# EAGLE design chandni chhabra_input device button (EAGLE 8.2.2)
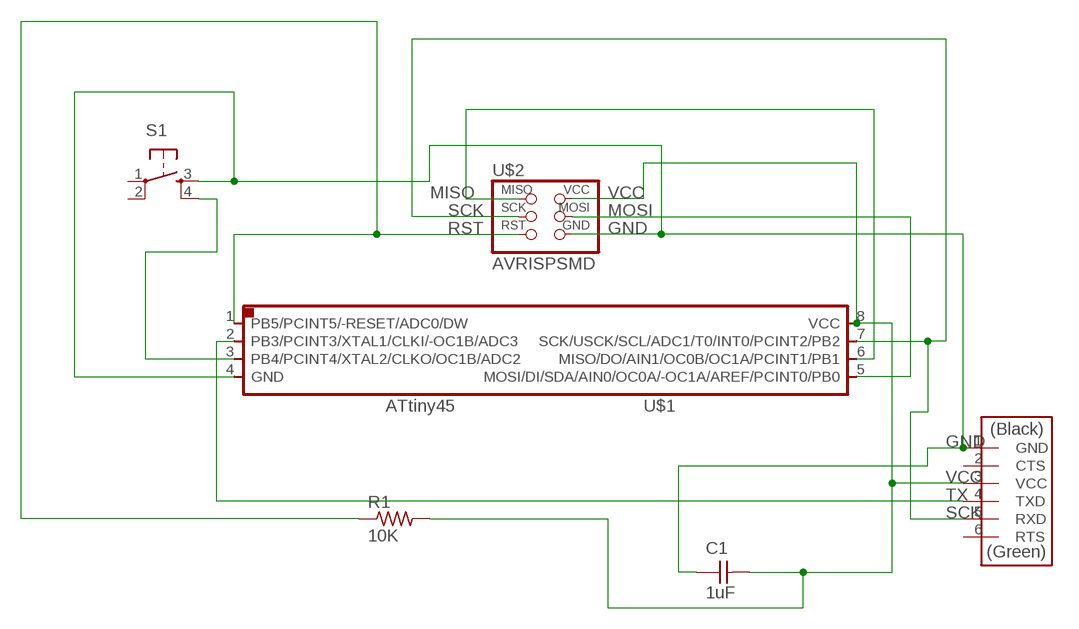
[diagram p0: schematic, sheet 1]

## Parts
C1  1uF  CAP-UNPOLARIZEDFAB  [C1206FAB]
R1  10K  RES-US1206FAB  [R1206FAB]
S1  6MM_SWITCH6MM_SWITCH  [6MM_SWITCH]
U$1  ATTINY45SI  [SOIC8]
U$2  AVRISPSMD  [2X03SMD]
U$3  FTDI-SMD-HEADER  [1X06SMD]

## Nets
GND: C1.1 S1.3(S) U$1.4(GND) U$2.6(GND) U$3.1(GND)
MISO: U$1.6(MISO/DO/AIN1/OC0B/OC1A/PCINT1/PB1) U$2.1(MISO)
MOSI: U$1.5(MOSI/DI/SDA/AIN0/OC0A/-OC1A/AREF/PCINT0/PB0) U$2.4(MOSI)
N$1: S1.4(S1) U$1.3(PB4/PCINT4/XTAL2/CLKO/OC1B/ADC2)
RST: R1.1 U$1.1(PB5/PCINT5/-RESET/ADC0/DW) U$2.5(RST)
SCK: U$1.7(SCK/USCK/SCL/ADC1/T0/INT0/PCINT2/PB2) U$2.3(SCK) U$3.5(RXD)
TX: U$1.2(PB3/PCINT3/XTAL1/CLKI/-OC1B/ADC3) U$3.4(TXD)
VCC: C1.2 R1.2 U$1.8(VCC) U$2.2(VCC) U$3.3(VCC)
Unconnected: S1.1(P) S1.2(P1) U$3.2(CTS) U$3.6(RTS)

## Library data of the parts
C1 = fab:CAP-UNPOLARIZED
R1 = fab:RES-US: Resistor (US Symbol)
S1 = fab:6MM_SWITCH: OMRON SWITCH
U$1 = fab:ATTINY45
U$2 = fab:AVRISP
U$3 = fab:FTDI-SMD-HEADER

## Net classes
0 default: width 0.32 mm, clearance 0.4 mm

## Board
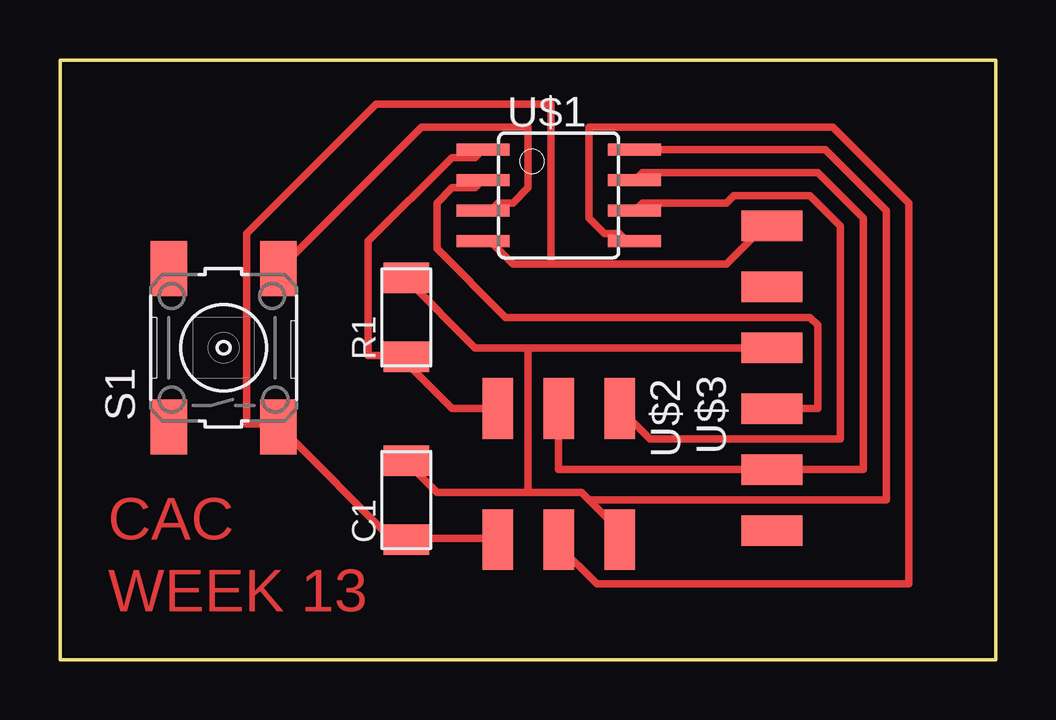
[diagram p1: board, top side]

Size 39 x 25 mm. Coordinates in mm from the lower left corner, seen from the top.
Outline: 39,25 0,25 0,0 39,0 39,25
Copper layers (1*16): Top 0.035mm / dielectric 1.5mm / Bottom 0.035mm
Design rules "fab": minimum track width 0.3mm, minimum drill 32mil, track to track 0.315mm, track to pad 0.315mm, pad to pad 0.315mm, via to via 0.315mm, smd to smd 0.315mm, copper to edge 40mil, drill to drill 16mil, minimum pad ring 10mil, minimum via ring 8mil, stop-mask expansion 4mil, vias tented up to drill 0mil, thermal gap 10mil

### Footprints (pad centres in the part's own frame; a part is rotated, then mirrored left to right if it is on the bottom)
C1206FAB = smd 1.27 x 1.905: 1 -1.651,0; 2 1.651,0
R1206FAB = smd 1.27 x 1.905: 1 -1.651,0; 2 1.651,0
6MM_SWITCH = smd 2.286 x 1.524: 1 -3.302,2.286; 2 3.302,2.286; 3 -3.302,-2.286; 4 3.302,-2.286
SOIC8 = smd 0.5 x 2.2: 1 -1.905,-3.154; 2 -0.645,-3.154; 3 0.625,-3.154; 4 1.895,-3.154; 5 1.905,3.154; 6 0.635,3.154; 7 -0.635,3.154; 8 -1.905,3.154
2X03SMD = smd 2.54 x 1.27: 1 -2.54,2.54; 2 2.92,2.54; 3 -2.54,0; 4 2.92,0; 5 -2.54,-2.54; 6 2.92,-2.54
1X06SMD = smd 2.54 x 1.27: 1 0,6.35; 2 0,3.81; 3 0,1.27; 4 0,-1.27; 5 0,-3.81; 6 0,-6.35

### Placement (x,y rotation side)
C1  14.44,6.65 90 top
R1  14.44,14.27 90 top
S1  6.82,13 90 top
U$1  20.79,19.35 270 top
U$2  20.79,7.92 270 top
U$3  29.68,11.73 0 top

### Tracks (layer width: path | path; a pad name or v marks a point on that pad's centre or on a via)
GND
  Top 0.32: 20.47,16.49 27.77,16.49 29.36,18.08 U$3.1 | 20.47,16.49 18.89,16.49 17.93,17.45 U$1.4 | 14.44,5.06 18.25,5.06 U$2.6 | 14.44,5.06 13.8,5.06 9.36,9.51 S1.3 9.04,9.82 7.77,9.82 7.77,17.76 13.17,23.16 20.47,23.16 20.47,16.49 | 14.44,5.06 C1.1
MISO
  Top 0.32: U$2.1 24.6,9.19 32.54,9.19 32.54,18.08 31.27,19.35 28.09,19.35 27.77,19.03 24.28,19.03 23.96,18.71 U$1.6
MOSI
  Top 0.32: U$1.5 23.65,17.45 23.33,17.76 22.7,17.76 22.06,18.4 22.06,22.21 32.22,22.21 35.39,19.03 35.39,3.16 22.38,3.16 20.79,4.74 U$2.4
N$1
  Top 0.32: U$1.3 17.93,18.71 18.25,19.03 18.89,19.03 19.52,19.67 19.52,22.21 15.08,22.21 9.36,16.49 S1.4
RST
  Top 0.32: U$2.5 16.34,10.46 14.44,12.37 R1.1 14.44,12.68 12.85,12.68 12.85,17.45 16.34,20.94 17.3,20.94 17.62,21.26 U$1.1
SCK
  Top 0.32: U$1.7 23.96,19.98 24.28,20.3 31.59,20.3 33.49,18.4 33.49,7.92 U$3.5 20.79,7.92 U$2.3
TX
  Top 0.32: U$3.4 31.59,10.46 31.59,13.95 31.27,14.27 18.57,14.27 15.71,17.13 15.71,19.03 16.34,19.67 17.3,19.67 17.62,19.98 U$1.2
VCC
  Top 0.32: U$3.3 19.52,13 | 19.52,13 17.3,13 14.44,15.86 R1.2 | 19.52,6.97 21.74,6.97 22.06,6.65 | 19.52,6.97 15.71,6.97 14.44,8.24 C1.2 | 22.06,6.65 23.33,5.38 U$2.2 | U$1.8 31.9,21.26 34.44,18.71 34.44,6.65 22.06,6.65 | 19.52,6.97 19.52,13

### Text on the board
Top: CAC | WEEK 13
